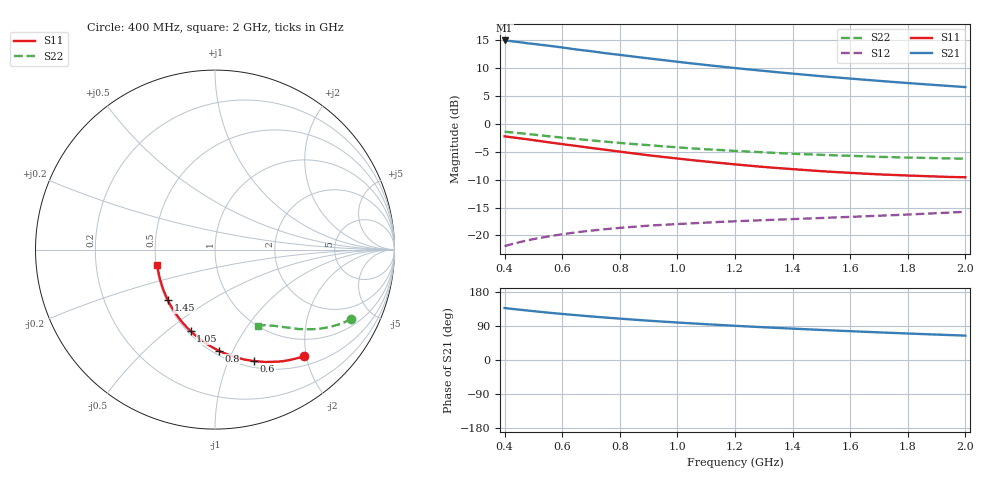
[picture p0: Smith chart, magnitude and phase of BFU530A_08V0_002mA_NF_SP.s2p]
! Filename:  P:\Prog\Test\Noise\ATS_data\Testdata_Net\06 Compressed Noise after Statistics\BFU530A_APG2013_33_A05_08p0V_002mA_NF_CM01_D.sf
! Date/Time: Tue 16/Apr/2013 15:10:56
! BFU530A_APG2013_33_A05_08p0V_1to25mA_NF_CM01_Bias2_R.sf
! Noise Parameter Data File
! BFU530A_APG2013_33_A05_08p0V_1to25mA_NF_CM01
! Date/time: Fri Apr 12 16:45:05 2013
! VAR V_out= 8.001000
! VAR I_out= 1.995000
! VAR V_in= 0.797000
! VAR I_in= 0.020100
! Device data file deembeded for feedlines and parallel
! Original file: \06 Compressed Noise after Statistics\BFU530A_APG2013_33_A05_08p0V_002mA_NF_CM01_R.sf
! Feed-files: PR017V01_150413_Feed1.s2p, PR017V01_150413_Feed2.s2p
! Parallel-file: PR017V01_150413_Par.s2p
# MHz S MA R 50
!  Freq-MHz  S11-mag  S11-arg  S21-mag  S21-arg  S12-mag  S12-arg  S22-mag  S22-arg
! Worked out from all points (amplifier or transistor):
!   37 points, 400 MHz to 2 GHz, reference 50 ohm
!   highest |S21| = 15.0 dB at 400 MHz (marker M1)
!   |S21| within 3 dB of that: start of sweep to 865.1 MHz
!   unconditionally stable (mu >= 1): nowhere
!   at 500 MHz: K = 0.34, MSG = 17.5 dB, |S12| = -20.7 dB
!   at 1.1 GHz: K = 0.68, MSG = 14.1 dB, |S12| = -17.7 dB
!   at 2 GHz: K = 0.99, MSG = 11.2 dB, |S12| = -15.8 dB
!   lowest NFmin = 0.48 dB at 420 MHz
!   S11 on the Smith chart (normalised r, x): 400 MHz: 0.66, -1.95; 600 MHz: 0.57, -1.25; 800 MHz: 0.53, -0.88; 1.05 GHz: 0.52, -0.61; 1.45 GHz: 0.51, -0.34; 2 GHz: 0.51, -0.10
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400  0.7733 -50.2  5.598 137.2  0.08018 62.0  0.8518 -26.9
420  0.7615 -52.5  5.529 135.3  0.08299 61.0  0.8417 -28.0
440  0.7498 -54.6  5.451 133.7  0.08558 60.1  0.8318 -28.9
480  0.7276 -58.7  5.279 130.5  0.09045 58.3  0.8114 -30.7
500  0.7151 -60.8  5.214 128.9  0.09278 57.5  0.8017 -31.5
550  0.6859 -65.9  5.032 125.1  0.09782 55.5  0.7762 -33.5
600  0.6586 -70.6  4.844 121.5  0.1025 53.9  0.7535 -35.3
650  0.6343 -75.0  4.645 118.3  0.1069 52.4  0.7332 -36.9
700  0.6089 -79.5  4.484 115.0  0.1104 51.1  0.7123 -38.5
750  0.5864 -83.6  4.305 112.0  0.1139 50.0  0.6934 -39.8
800  0.5644 -87.8  4.157 109.2  0.1169 49.0  0.6758 -41.0
850  0.5432 -91.8  4.005 106.4  0.1197 48.2  0.659 -42.2
950  0.5057 -99.5  3.735 101.3  0.1244 46.9  0.6292 -44.4
1050  0.4739 -106.6  3.485 96.6  0.1285 46.1  0.6034 -46.3
1100  0.4599 -110.2  3.373 94.5  0.1304 45.9  0.5923 -47.1
1200  0.4338 -117.0  3.169 90.3  0.1339 45.5  0.5728 -48.8
1300  0.4112 -123.5  2.988 86.4  0.1371 45.5  0.5561 -50.4
1450  0.3849 -133.1  2.749 81.0  0.1418 46.0  0.5341 -52.6
1500  0.377 -136.3  2.677 79.3  0.1434 46.2  0.5282 -53.3
1650  0.3582 -145.2  2.489 74.5  0.1485 47.3  0.5125 -55.5
1750  0.3488 -151.1  2.376 71.4  0.1521 48.2  0.5033 -56.9
2000  0.3327 -164.8  2.139 64.3  0.163 50.6  0.4878 -60.7
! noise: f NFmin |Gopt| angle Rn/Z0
400  0.4978  0.5402  20.68  0.2016
460  0.5235  0.5167  29.47  0.1916
600  0.5825  0.4871  34.06  0.2064
800  0.6047  0.4475  48.6  0.1663
1000  0.5898  0.4255  62.25  0.1597
1200  0.7106  0.4191  75.2  0.1476
1400  0.7639  0.4013  91.01  0.12
1600  0.8009  0.3847  103.6  0.1033
1800  0.7228  0.3809  127.3  0.0765
2000  0.7928  0.4278  133.1  0.0639
